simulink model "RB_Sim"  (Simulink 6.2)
settings: Solver=ode4  StartTime=0.0  StopTime=2000  FixedStep=Tsr  MaxStep=0.000001  RelTol=1e-12  AbsTol=1e-8
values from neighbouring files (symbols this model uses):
  Cw2b = [ 0,          0,          0    [start.m]    (also in run.m)
  d2r = pi/180    (= 0.0174532925199)    [start.m]    (also in run.m; runf.m; orbitic.m; Quan.m)
  Hmax = 10    [start.m]    (also in run.m)
  Jw = [Iw, 0, 0    [start.m]    (also in run.m)
  Kq1 = I22*ww^2 - 3*wo2*(I11-I33)    [start.m]    (also in run.m)
  Kq2 = 2*I22*zet*ww    [start.m]    (also in run.m)
  Kqi = 0.0005    [start.m]    (also in run.m)
  Kr1 = (0.1*I11*I33*zet^2/Hy0) - sqrt( ((0.01^zet^4*I11^2*I33^2)/Hy0^2)+(4*I11*I33*zet^2) )    [start.m]    (also in run.m)
  Kr2 = 0.05*Kr1    [start.m]    (also in run.m)
  Kr3 = 0.04*zet*(Kr2-Hy0) * sqrt(abs(Hy0/(I11*I33)))    [start.m]    (also in run.m)
  nt = 7    [start.m]    (also in run.m; runf.m)
  r2d = 180/pi    (= 57.2957795131)    [pl.m]    (also in pld.m; start.m; run.m; plf.m)
  Tmax = 0.05    [start.m]    (also in run.m)
  Ts = 0.01    [start.m]    (also in run.m = 0.001; runf.m = 0.0005)
  wo = 0.00113    [start.m]    (also in run.m)
undefined symbols (not defined in the file or in its folder): Arb, Brb, Crb, den, DiscIntNeverNeededParam, Drb, dsen, nsen, num, Phase_Plane, RW_Steering
libraries: simulink x7

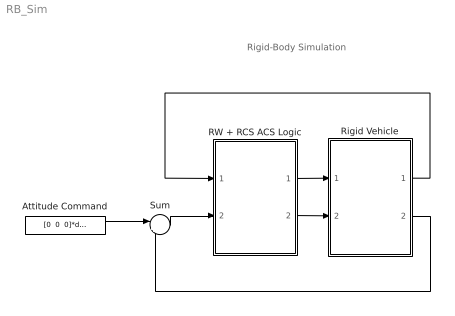
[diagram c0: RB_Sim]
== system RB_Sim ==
  note: Rigid-Body Simulation
  Attitude Command : Constant  Value="[0  0  0]*d2r"
  RW + RCS ACS Logic : Subsystem
  Rigid Vehicle : Subsystem
  Sum : Sum  Inputs=|+-
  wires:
  Attitude Command/1 -> Sum/1
  Sum/1 -> RW + RCS ACS Logic/2(atter)
  Rigid Vehicle/2(atti) -> Sum/2
  Rigid Vehicle/1(Wr) -> RW + RCS ACS Logic/1(wr(i))
  RW + RCS ACS Logic/1(Frcs) -> Rigid Vehicle/1(Thr7)
  RW + RCS ACS Logic/2(Trwi) -> Rigid Vehicle/2(Trw(i))

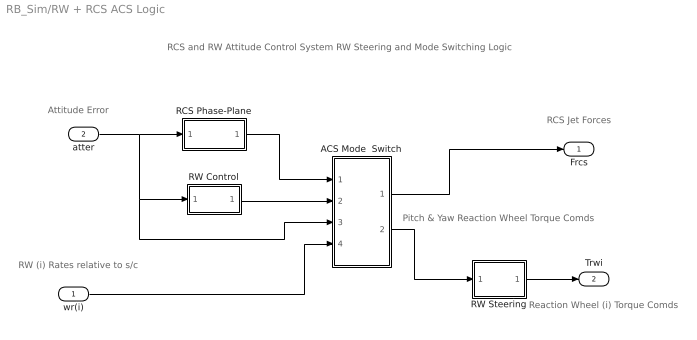
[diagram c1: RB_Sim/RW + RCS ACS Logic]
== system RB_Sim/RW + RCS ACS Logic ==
  note: RCS and RW Attitude Control System RW Steering and Mode Switching Logic
  note: RCS Jet Forces
  note: Reaction Wheel (i) Torque Comds
  note: RW (i) Rates relative to s/c
  note: Attitude Error
  note: Pitch & Yaw Reaction Wheel Torque Comds
  wr(i) : Inport  Port=1  LatchInput=off
  atter : Inport  Port=2  LatchInput=off
  ACS Mode  Switch : Subsystem
  RCS Phase-Plane : Subsystem
  RW Control : Subsystem
  RW Steering : Subsystem
  Frcs : Outport
  Trwi : Outport  Port=2
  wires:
  atter/1 -> RCS Phase-Plane/1(atter), ACS Mode  Switch/3(atter), RW Control/1(atti)
  RW Control/1(Tc) -> ACS Mode  Switch/2(Trw)
  ACS Mode  Switch/2(" Trw") -> RW Steering/1(Trwc)
  wr(i)/1 -> ACS Mode  Switch/4(wr(i))
  RCS Phase-Plane/1(f(nt)) -> ACS Mode  Switch/1(Frcs)
  RW Steering/1(Twi) -> Trwi/1
  ACS Mode  Switch/1(" Frcs") -> Frcs/1

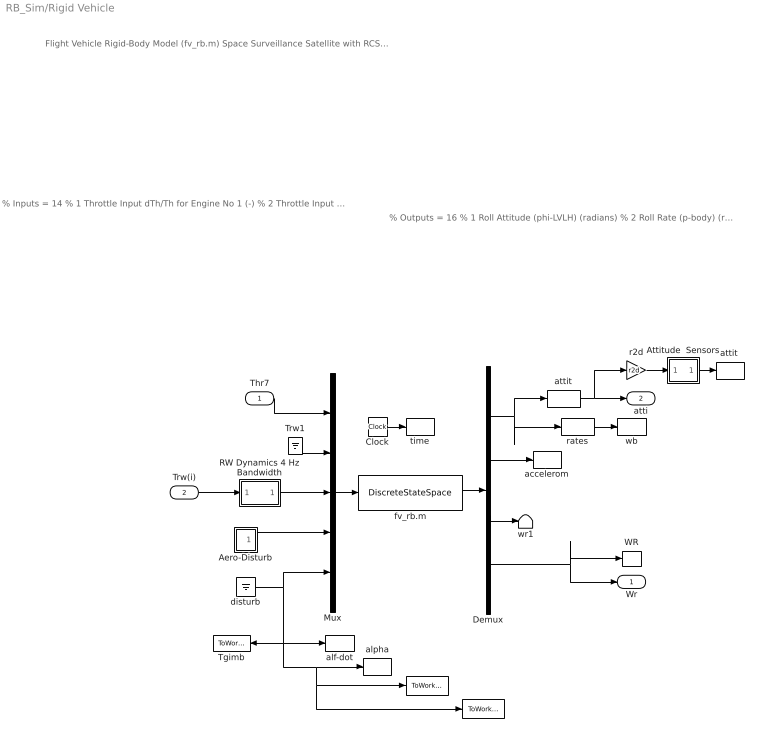
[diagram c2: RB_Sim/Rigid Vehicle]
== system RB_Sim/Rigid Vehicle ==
  note: % Inputs = 14 % 1 Throttle Input dTh/Th for Engine No 1 (-) % 2 Throttle Input dTh/Th for Engine No 2 (-) % 3 Throttle Input dTh/Th for Engine No 3 (-) % 4 Throttle Input dTh/Th for Engine No 4 (-) % 5 Throttle Input dTh/Th for Engine No 5 (-) % 6 Throttle Input dTh/Th for Engine No 6 (-) % 7 Throttle Input dTh/Th for Engine No 7 (-) % 8 Reaction Wheel No 1 Input Torque (ft-lb) % 9 Reaction Wheel No 2 Input Torque (ft-lb) % 10 Reaction Wheel No 3 Input Torque (ft-lb) % 11 Ext Torque Input 1 (ft-lb), dir: 1.00 0.00 0.00 % 12 Ext Torque Input 2 (ft-lb), dir: 0.00 1.00 0.00 % 13 Ext Torque Input 3 (ft-lb), dir: 0.00 0.00 1.00 % 14 Ext Torque Direct.=( 0.1970 -0.5964 -0.7782)
  note: % Outputs = 16 % 1 Roll Attitude (phi-LVLH) (radians) % 2 Roll Rate (p-body) (rad/sec) % 3 Pitch Attitude (thet-LVLH) (radians) % 4 Pitch Rate (q-body) (rad/sec) % 5 Yaw Attitude (psi-LVLH) (radians) % 6 Yaw Rate (r-body) (rad/sec) % 7 Angle of attack, alfa, (radians) % 8 Angle of sideslip, beta, (radian) % 9 Change in Altitude, delta-h, (feet) % 10 Forward Acceleration (V-dot) (ft/sec) % 11 Cross Range Velocity (Vcr) (ft/sec) % 12 Accelerom # 1, (along X), (ft/sec^2) Translat. Acceler % 13 Accelerom # 2, (along Y), (ft/sec^2) Translat. Acceler % 14 Reaction Wheel # 1 Rate (rpm) relative to vehicle % 15 Reaction Wheel # 2 Rate (rpm) relative to vehicle % 16 Reaction Wheel # 3 Rate (rpm) relative to vehicle
  note: Flight Vehicle Rigid-Body Model (fv_rb.m) Space Surveillance Satellite with RCS and Reaction Wheels (Rigid-Body)
  Thr7 : Inport  Port=1  LatchInput=off
  Trw(i) : Inport  Port=2  LatchInput=off
  " " : ToWorkspace  VariableName=SA_pos  SampleTime=-1  SaveFormat=Array
  "   " : ToWorkspace  VariableName=SA_rate  SampleTime=-1  SaveFormat=Array
  Aero-Disturb : Subsystem
  Attitude  Sensors : Subsystem
  Clock : Clock
  Demux : Demux  Outputs=[11, 2, 1,2]
  Mux : Mux  Inputs=[7, 1,2, 3, 1]
  RW Dynamics 4 Hz Bandwidth : Subsystem
  Tgimb : ToWorkspace  VariableName=Tgimb  SampleTime=-1  SaveFormat=Array
  Trw1 : Ground
  WR : ToWorkspace  VariableName=wr  SampleTime=-1  SaveFormat=Array
  accelerom : ToWorkspace  VariableName=accel  SampleTime=-1  SaveFormat=Array
  alf-dot : ToWorkspace  VariableName=alfad  SampleTime=-1  SaveFormat=Array
  alpha : ToWorkspace  VariableName=alfa  SampleTime=-1  SaveFormat=Array
  attit : Selector  Elements=[1, 3, 5]  InputPortWidth=11
  "attit " : ToWorkspace  VariableName=atti  SampleTime=-1  SaveFormat=Array
  disturb : Ground
  fv_rb.m : DiscreteStateSpace  A=Arb  B=Brb  C=Crb  D=Drb  SampleTime=Ts
  r2d : Gain  Gain=r2d
  rates : Selector  Elements=[2, 4, 6]  InputPortWidth=11
  time : ToWorkspace  VariableName=time  SampleTime=-1  SaveFormat=Array
  wb : ToWorkspace  VariableName=wb  SampleTime=-1  SaveFormat=Array
  wr1 : Terminator
  Wr : Outport
  atti : Outport  Port=2
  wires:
  Thr7/1 -> Mux/1
  Trw(i)/1 -> RW Dynamics 4 Hz Bandwidth/1(I)
  Demux/1 -> attit/1, rates/1
  attit/1 -> atti/1, r2d/1
  Demux/4 -> Wr/1, WR/1
  disturb/1 -> alf-dot/1, alpha/1, "   "/1, " "/1, Tgimb/1, Mux/5
  rates/1 -> wb/1
  r2d/1 -> Attitude  Sensors/1(I)
  Aero-Disturb/1(Td) -> Mux/4
  Clock/1 -> time/1
  Mux/1 -> fv_rb.m/1
  fv_rb.m/1 -> Demux/1
  Demux/2 -> accelerom/1
  Trw1/1 -> Mux/2
  Demux/3 -> wr1/1
  RW Dynamics 4 Hz Bandwidth/1(O) -> Mux/3
  Attitude  Sensors/1(O) -> "attit "/1

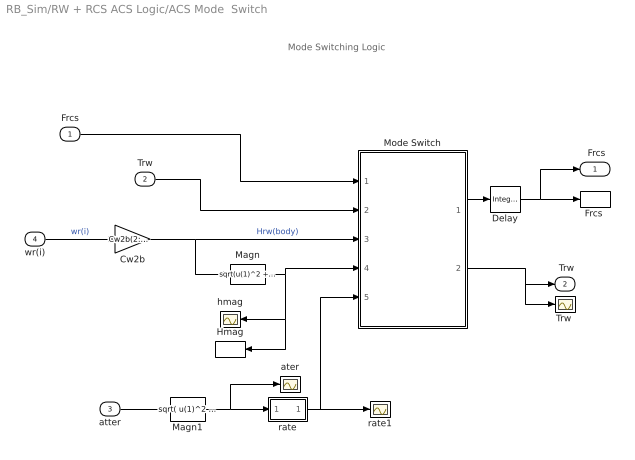
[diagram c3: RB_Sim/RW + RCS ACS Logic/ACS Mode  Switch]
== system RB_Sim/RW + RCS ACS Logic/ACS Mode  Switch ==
  note: Mode Switching Logic
  Frcs : Inport  Port=1  LatchInput=off
  Trw : Inport  Port=2  LatchInput=off
  atter : Inport  Port=3  LatchInput=off
  wr(i) : Inport  Port=4  LatchInput=off
  Cw2b : Gain  Gain=Cw2b(2:3,2:3)*Jw(2:3,2:3)  Multiplication=Matrix(K*u)
  Delay : simulink/Discrete/Integer Delay  vinit=0.0  samptime=Tsr  NumDelays=1
  "Frcs " : ToWorkspace  VariableName=Frcs  SampleTime=-1  SaveFormat=Array
  Hmag : ToWorkspace  VariableName=Hmag  SampleTime=-1  SaveFormat=Array
  Magn : Fcn  Expr=sqrt(u(1)^2 + u(2)^2)
  Magn1 : Fcn  Expr=sqrt( u(1)^2 + u(2)^2 + u(3)^2 )
  Mode Switch : Stateflow chart
  "Trw " : Scope
  ater : Scope
  hmag : Scope
  rate : Subsystem
  rate1 : Scope
  " Frcs" : Outport
  " Trw" : Outport  Port=2
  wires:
  wr(i)/1 -> Cw2b/1  "wr(i)"
  Frcs/1 -> Mode Switch/1(Fi)
  Trw/1 -> Mode Switch/2(Tci)
  atter/1 -> Magn1/1
  Magn/1 -> Mode Switch/4(hmag), hmag/1, Hmag/1
  Mode Switch/1(Fo) -> Delay/1
  Mode Switch/2(Tco) -> " Trw"/1, "Trw "/1
  Cw2b/1 -> Mode Switch/3(hrwa), Magn/1  "Hrw(body)"
  Magn1/1 -> rate/1(in), ater/1
  rate/1(ou) -> Mode Switch/5(atter), rate1/1
  Delay/1 -> "Frcs "/1, " Frcs"/1

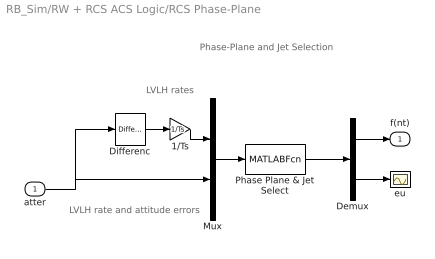
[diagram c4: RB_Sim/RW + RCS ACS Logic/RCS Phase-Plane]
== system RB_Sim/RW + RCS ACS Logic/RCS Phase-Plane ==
  note: Phase-Plane and Jet Selection
  note: LVLH rate and attitude errors
  note: LVLH rates
  atter : Inport  Port=1  LatchInput=off
  1/Ts : Gain  Gain=1/Ts
  Demux : Demux  Outputs=[nt, 3]
  Differenc : simulink/Discrete/Difference  ICPrevInput=0.0  OutDataType=sfix(16)  OutScaling=2^-10  DoSatur=off
  Mux : Mux  Inputs="[3  3]"
  Phase Plane & Jet Select : MATLABFcn  MATLABFcn=Phase_Plane( u(1:3), u(4:6) )  OutputDimensions=nt + 3
  eu : Scope
  f(nt) : Outport
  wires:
  atter/1 -> Mux/2, Differenc/1
  1/Ts/1 -> Mux/1
  Demux/2 -> eu/1
  Demux/1 -> f(nt)/1
  Phase Plane & Jet Select/1 -> Demux/1
  Mux/1 -> Phase Plane & Jet Select/1
  Differenc/1 -> 1/Ts/1

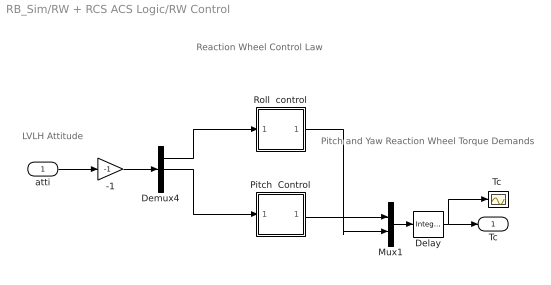
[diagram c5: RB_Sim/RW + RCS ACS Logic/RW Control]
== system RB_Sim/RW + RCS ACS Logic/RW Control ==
  note: Reaction Wheel Control Law
  note: LVLH Attitude
  note: Pitch and Yaw Reaction Wheel Torque Demands
  atti : Inport  Port=1  LatchInput=off
  -1 : Gain  Gain=-1
  Delay : simulink/Discrete/Integer Delay  vinit=0.0  samptime=Tsr  NumDelays=1
  Demux4 : Demux  Outputs=3
  Mux1 : Mux  Inputs=2
  Pitch  Control : Subsystem
  Roll  control : Subsystem
  "Tc " : Scope
  Tc : Outport
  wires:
  Roll  control/1(Tcz) -> Mux1/2
  -1/1 -> Demux4/1
  Mux1/1 -> Delay/1
  atti/1 -> -1/1
  Demux4/2 -> Pitch  Control/1(the)
  Pitch  Control/1(Tcy) -> Mux1/1
  Demux4/1 -> Roll  control/1(phi)
  Delay/1 -> Tc/1, "Tc "/1

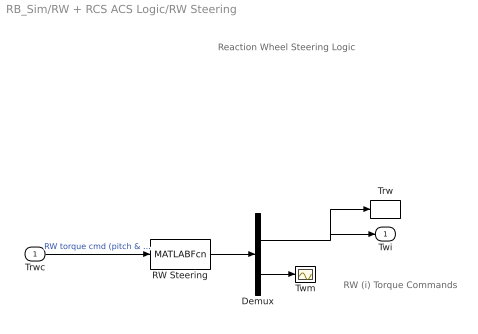
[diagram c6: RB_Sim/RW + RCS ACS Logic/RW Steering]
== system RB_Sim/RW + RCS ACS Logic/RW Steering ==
  note: RW (i) Torque Commands
  note: Reaction Wheel Steering Logic
  Trwc : Inport  Port=1  LatchInput=off
  Demux : Demux  Outputs=[2, 1]
  RW Steering : MATLABFcn  MATLABFcn=RW_Steering( u(1:2) )  OutputDimensions=3
  Trw : ToWorkspace  VariableName=Trw  SampleTime=-1  SaveFormat=Array
  Twm : Scope
  Twi : Outport
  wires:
  Demux/2 -> Twm/1
  Demux/1 -> Twi/1, Trw/1
  RW Steering/1 -> Demux/1
  Trwc/1 -> RW Steering/1  "RW torque cmd (pitch & yaw)"

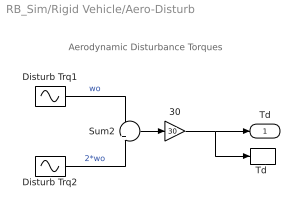
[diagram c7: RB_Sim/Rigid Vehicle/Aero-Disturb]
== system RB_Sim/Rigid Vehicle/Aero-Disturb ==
  note: Aerodynamic Disturbance Torques
  30 : Gain  Gain=30
  Disturb Trq1 : Sin  Amplitude="[0.0,   1,   0.2]*0.0001"  Bias="[0.0,  0.5,  0.15]*0.0001"  Frequency=[wo, wo, wo]  SampleTime=0
  Disturb Trq2 : Sin  Amplitude=[0, 1.2, 1]*0.0001  Bias=[0 0 0]  Frequency=[wo, wo, wo]*2  SampleTime=0
  Sum2 : Sum  Inputs=+|+
  "Td " : ToWorkspace  VariableName=Td  SampleTime=-1  SaveFormat=Array
  Td : Outport
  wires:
  30/1 -> "Td "/1, Td/1
  Disturb Trq2/1 -> Sum2/2  "2*wo"
  Sum2/1 -> 30/1
  Disturb Trq1/1 -> Sum2/1  "wo"

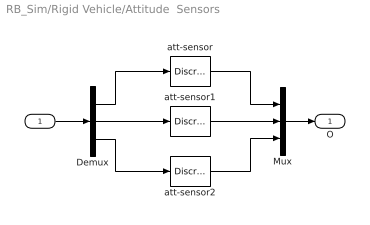
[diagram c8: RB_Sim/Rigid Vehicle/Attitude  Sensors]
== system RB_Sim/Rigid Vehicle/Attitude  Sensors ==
  I : Inport  Port=1  LatchInput=off
  Demux : Demux  Outputs=3
  Mux : Mux  Inputs=3
  att-sensor : DiscreteTransferFcn  Numerator=[nsen]  Denominator=[dsen]  SampleTime=Ts
  att-sensor1 : DiscreteTransferFcn  Numerator=[nsen]  Denominator=[dsen]  SampleTime=Ts
  att-sensor2 : DiscreteTransferFcn  Numerator=[nsen]  Denominator=[dsen]  SampleTime=Ts
  O : Outport
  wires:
  I/1 -> Demux/1
  Mux/1 -> O/1
  att-sensor/1 -> Mux/1
  Demux/1 -> att-sensor/1
  Demux/3 -> att-sensor2/1
  att-sensor2/1 -> Mux/3
  Demux/2 -> att-sensor1/1
  att-sensor1/1 -> Mux/2

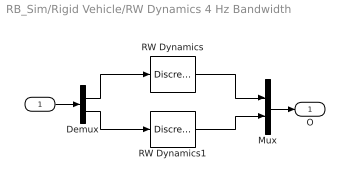
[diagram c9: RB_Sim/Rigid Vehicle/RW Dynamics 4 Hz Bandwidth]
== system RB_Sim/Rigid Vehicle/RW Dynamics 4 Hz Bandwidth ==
  I : Inport  Port=1  LatchInput=off
  Demux : Demux  Outputs=2
  Mux : Mux  Inputs=2
  RW Dynamics : DiscreteTransferFcn  Numerator="[0  0.221199217]"  Denominator=[1 -0.778800783]  SampleTime=Ts
  RW Dynamics1 : DiscreteTransferFcn  Numerator="[0  0.221199217]"  Denominator=[1 -0.778800783]  SampleTime=Ts
  O : Outport
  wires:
  Demux/2 -> RW Dynamics1/1
  Demux/1 -> RW Dynamics/1
  I/1 -> Demux/1
  Mux/1 -> O/1
  RW Dynamics/1 -> Mux/1
  RW Dynamics1/1 -> Mux/2

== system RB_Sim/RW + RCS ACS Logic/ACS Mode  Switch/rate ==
  in : Inport  Port=1  LatchInput=off
  1/Ts : Gain  Gain=1/Ts
  Abs : Abs
  Differenc : simulink/Discrete/Difference  ICPrevInput=0.0  OutDataType=sfix(16)  OutScaling=2^-10  DoSatur=off
  ou : Outport
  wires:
  Differenc/1 -> 1/Ts/1
  1/Ts/1 -> Abs/1
  in/1 -> Differenc/1
  Abs/1 -> ou/1

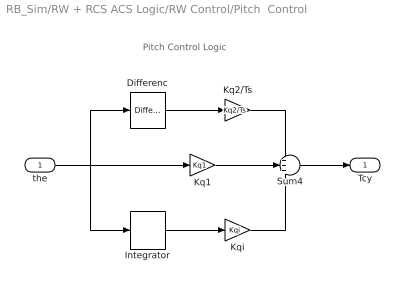
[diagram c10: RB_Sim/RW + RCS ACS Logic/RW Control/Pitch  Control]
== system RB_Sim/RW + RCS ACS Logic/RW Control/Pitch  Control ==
  note: Pitch Control Logic
  the : Inport  Port=1  LatchInput=off
  Differenc : simulink/Discrete/Difference  ICPrevInput=0.0  OutDataType=sfix(16)  OutScaling=2^-10  DoSatur=off
  Integrator : DiscreteIntegrator  SampleTime=Ts  ICPrevOutput=DiscIntNeverNeededParam  ICPrevScaledInput=DiscIntNeverNeededParam
  Kq1 : Gain  Gain=Kq1
  Kq2/Ts : Gain  Gain=Kq2/Ts
  Kqi : Gain  Gain=Kqi
  Sum4 : Sum  Inputs=+++
  Tcy : Outport
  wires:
  Differenc/1 -> Kq2/Ts/1
  Integrator/1 -> Kqi/1
  Kqi/1 -> Sum4/3
  the/1 -> Differenc/1, Integrator/1, Kq1/1
  Kq2/Ts/1 -> Sum4/1
  Sum4/1 -> Tcy/1
  Kq1/1 -> Sum4/2

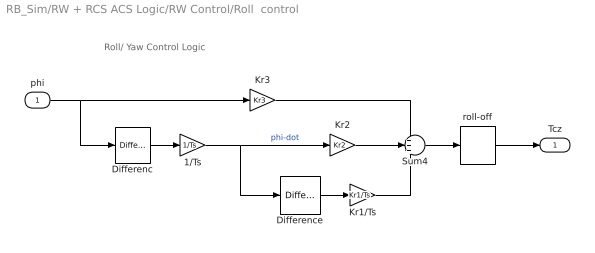
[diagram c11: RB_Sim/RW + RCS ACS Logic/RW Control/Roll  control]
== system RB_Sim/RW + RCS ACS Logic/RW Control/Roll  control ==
  note: Roll/ Yaw Control Logic
  phi : Inport  Port=1  LatchInput=off
  1/Ts : Gain  Gain=1/Ts
  Differenc : simulink/Discrete/Difference  ICPrevInput=0.0  OutDataType=sfix(16)  OutScaling=2^-10  DoSatur=off
  Difference : simulink/Discrete/Difference  ICPrevInput=0.0  OutDataType=sfix(16)  OutScaling=2^-10  DoSatur=off
  Kr1/Ts : Gain  Gain=Kr1/Ts
  Kr2 : Gain  Gain=Kr2
  Kr3 : Gain  Gain=Kr3
  Sum4 : Sum  Inputs=+++
  roll-off : DiscreteTransferFcn  Numerator=[num]  Denominator=[den]  SampleTime=Ts
  Tcz : Outport
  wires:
  1/Ts/1 -> Difference/1, Kr2/1  "phi-dot"
  Differenc/1 -> 1/Ts/1
  Difference/1 -> Kr1/Ts/1
  Sum4/1 -> roll-off/1
  phi/1 -> Differenc/1, Kr3/1
  Kr1/Ts/1 -> Sum4/3
  Kr2/1 -> Sum4/2
  Kr3/1 -> Sum4/1
  roll-off/1 -> Tcz/1

== stateflow chart RW + RCS
ACS Logic/ACS Mode 
Switch/Mode
Switch ==
  state RCS1
    en:Fo=Fi;
    en:Tco=-hrwa*Tmax/hmag;
  state RW
    en:Fo=Fz;
    en:Tco=Tci;
  state RCS2
    en:Fo=Fi;
    en:Tco=Tz;
  RW -> RCS1 : [hmag>=Hmax]
  RCS1 -> RCS1 : [hmag>=Hmax/10 ... || atter>=Rlim]
  (default) -> RW
  RW -> RW : [hmag<Hmax]
  (junction 6) -> RW : [hmag<Hmax/10 ... && atter<Rlim]
  RCS1 -> (junction 6)
  (junction 6) -> RCS2
  RCS2 -> RW : [atter<Rlim]
  RCS2 -> RCS1 : [hmag>Hmax/10]
